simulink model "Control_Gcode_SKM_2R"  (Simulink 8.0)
settings: Solver=FixedStepDiscrete  SolverMode=SingleTasking  StartTime=0  StopTime=inf  FixedStep=dt  RelTol=1e-3  SampleTimeConstraint=Specified
InitFcn:
  | % Sampling Times %
  | dt0=0.001; dt1=0.01; samples=10;
undefined symbols (not defined in the file or in its folder): DiscIntNeverNeededParam, Volts
libraries: simulink_extras x4, speedgoatlib_IO311 x3, xpclib x3, speedgoatlib_IO101 x2, simulink x2

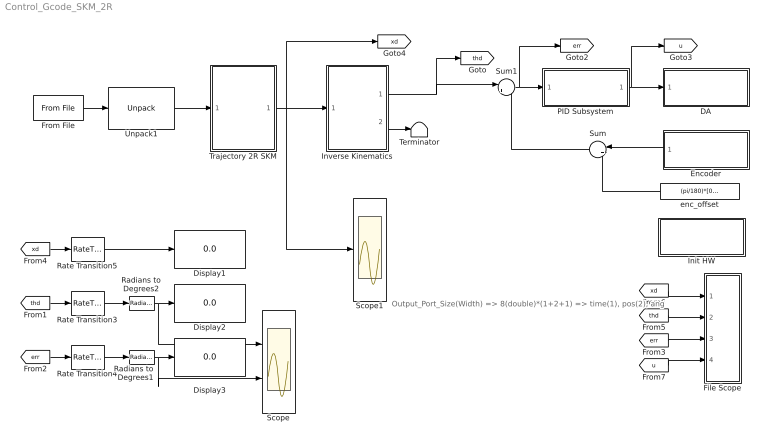
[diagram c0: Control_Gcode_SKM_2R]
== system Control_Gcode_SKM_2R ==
  note: Output_Port_Size(Width) => 8(double)*(1+2+1) => time(1), pos(2), ang
  DA : Subsystem  TreatAsAtomicUnit=on
  Display1 : Display
  Display2 : Display
  Display3 : Display
  Encoder : Subsystem  TreatAsAtomicUnit=on
  File Scope : Subsystem
  From File : xpclib/Misc./From File  filename='skm1.dat'  dataSize=32  bufSize=4000  readSize=1024  EOFOption=Hold last output  sampTime=dt0  show2ports=off
  Init HW : Subsystem  TreatAsAtomicUnit=on
  Inverse Kinematics : MATLAB Function  TreatAsAtomicUnit=on
  PID Subsystem : Subsystem  TreatAsAtomicUnit=on
  Radians to Degrees1 : simulink_extras/Transformations/Radians to Degrees
  Radians to Degrees2 : simulink_extras/Transformations/Radians to Degrees
  Rate Transition3 : RateTransition  OutPortSampleTime=dt1
  Rate Transition4 : RateTransition  OutPortSampleTime=dt1
  Rate Transition5 : RateTransition  OutPortSampleTime=dt1
  Scope : Scope  NumInputPorts=2
  Scope1 : Scope
  Sum : Sum  Inputs=|++
  Sum1 : Sum  Inputs=|+-
  Terminator : Terminator
  Trajectory 2R SKM : MATLAB Function  TreatAsAtomicUnit=on
  Unpack1 : xpclib/UDP/Unpack  dimensions={[4]}  datatypes={'double'}  byteAlign=1
  enc_offset : Constant  Value=(pi/180)*[0,90]'
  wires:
  [thd] -> Rate Transition3/1
  [err] -> Rate Transition4/1
  [xd] -> Rate Transition5/1
  Rate Transition5/1 -> Display1/1
  Rate Transition3/1 -> Radians to Degrees2/1
  Rate Transition4/1 -> Radians to Degrees1/1
  Radians to Degrees2/1 -> Display2/1, Scope/1
  Radians to Degrees1/1 -> Display3/1, Scope/2
  [xd] -> File Scope/1(xd)
  [thd] -> File Scope/2(thd)
  [err] -> File Scope/3(err)
  [u] -> File Scope/4(u)
  From File/1 -> Unpack1/1
  Sum1/1 -> PID Subsystem/1(In1), [err]
  PID Subsystem/1(Out1) -> DA/1(In1), [u]
  Encoder/1(Out1) -> Sum/1
  enc_offset/1 -> Sum/2
  Sum/1 -> Sum1/2
  Trajectory 2R SKM/1(xd) -> [xd], Inverse Kinematics/1(xd), Scope1/1
  Inverse Kinematics/1(thd) -> Sum1/1, [thd]
  Inverse Kinematics/2(w_index) -> Terminator/1
  Unpack1/1 -> Trajectory 2R SKM/1(traj)

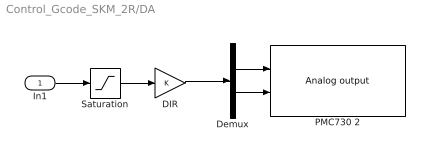
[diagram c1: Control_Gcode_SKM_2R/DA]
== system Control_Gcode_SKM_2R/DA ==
  In1 : Inport
  DIR : Gain
  Demux : Demux  Outputs=2
  PMC730 2 : speedgoatlib_IO101/Analog output  id=1  channel=[1,2]  reset=[1,1]  initValue=[0,0]  ts=dt0  pciSlot=-1
  Saturation : Saturate  UpperLimit=10  LowerLimit=-10
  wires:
  In1/1 -> Saturation/1
  Saturation/1 -> DIR/1
  DIR/1 -> Demux/1
  Demux/2 -> PMC730 2/2
  Demux/1 -> PMC730 2/1

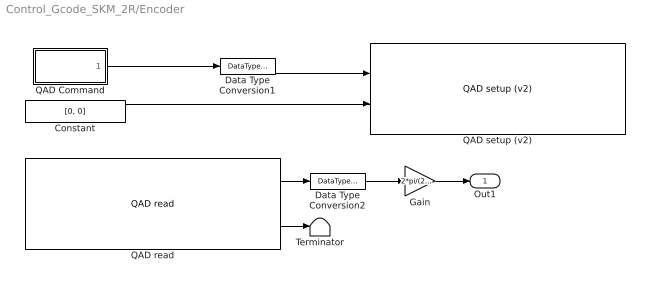
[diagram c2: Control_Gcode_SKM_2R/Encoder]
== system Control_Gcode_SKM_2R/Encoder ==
  Constant : Constant  Value=[0, 0]  OutDataTypeStr=Inherit: Inherit via back propagation
  Data Type Conversion1 : DataTypeConversion  OutDataTypeStr=uint8
  Data Type Conversion2 : DataTypeConversion  OutDataTypeStr=double
  Gain : Gain  Gain=2*pi/(23*2000)
  QAD Command : MATLAB Function  TreatAsAtomicUnit=on
  QAD read : speedgoatlib_IO311/QAD/QAD read  id=1  chan=[1 2]  pciSlot=-1  ts=dt0
  QAD setup (v2) : speedgoatlib_IO311/QAD/QAD setup (v2)  id=1  chan=[1,2]  debounce=0  quadrature=4x  index=Ignore index input  special=Disabled (cycling counter)  steps=2000  ts=dt0  pciSlot=-1
  Terminator : Terminator
  Out1 : Outport
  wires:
  Gain/1 -> Out1/1
  Constant/1 -> QAD setup (v2)/2
  QAD read/2 -> Terminator/1
  QAD read/1 -> Data Type Conversion2/1
  QAD Command/1(y) -> Data Type Conversion1/1
  Data Type Conversion2/1 -> Gain/1
  Data Type Conversion1/1 -> QAD setup (v2)/1

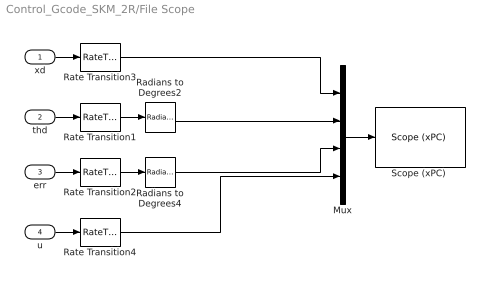
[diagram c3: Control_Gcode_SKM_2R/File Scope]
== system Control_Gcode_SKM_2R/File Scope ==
  xd : Inport
  thd : Inport  Port=2
  err : Inport  Port=3
  u : Inport  Port=4
  Mux : Mux
  Radians to Degrees2 : simulink_extras/Transformations/Radians to Degrees
  Radians to Degrees4 : simulink_extras/Transformations/Radians to Degrees
  Rate Transition{1..4} (4 alike) : RateTransition  OutPortSampleTime=dt1
  "Scope (xPC) " : xpclib/Misc./Scope (xPC)   scopeno=2  scopetype=File  autostart=on  viewmode=Graphical redraw  formatstr='%15.6f'  grid=on  ylimits=[0,0]  nosamples=100  noprepostsamples=0  interleave=1  triggermode=FreeRun  triggersignal=1  triggerlevel=0.0  triggerslope=Either  triggerscope=1  triggersample=0  filename=step3.dat  mode=Lazy  writesize=512  autorestart=on  dynamicfilemode=off  maxwritefilesize=512*1024^2
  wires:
  Radians to Degrees2/1 -> Mux/2
  Radians to Degrees4/1 -> Mux/3
  Rate Transition1/1 -> Radians to Degrees2/1
  Rate Transition2/1 -> Radians to Degrees4/1
  thd/1 -> Rate Transition1/1
  err/1 -> Rate Transition2/1
  Rate Transition3/1 -> Mux/1
  xd/1 -> Rate Transition3/1
  u/1 -> Rate Transition4/1
  Mux/1 -> "Scope (xPC) "/1
  Rate Transition4/1 -> Mux/4

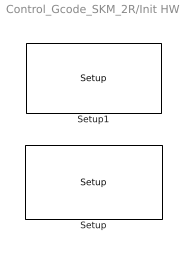
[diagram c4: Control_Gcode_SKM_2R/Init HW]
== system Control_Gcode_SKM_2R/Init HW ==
  Setup : speedgoatlib_IO311/Setup/Setup  group=Module setup  id=1  fpga1=speedgoat_IO311_default  pciSlot=-1  lowerDirection=[1 1 1 1 1 0 0 0 0 0 0 0 1 0 0 0]  lowerReset=[1]  lowerValue=[0]  upperDirection=[1 1 1 1 1 1 1 1 1 0 0 0 0 0 0 0]  upperReset=[1]  upperValue=[0]
  Setup1 : speedgoatlib_IO101/Setup  group=Module setup  id=1  pciSlot=-1  adStartChannel=1  adNumChannel=32  adCoupling=Single-ended  adRange=-10 .. 10 Volts  adAcqMode=Standard  daChannel=[1,2]  daReset=[1,1]  daInitValue=[0,0]  lowerChannel=1  lowerDirection=Input  lowerDIDebounce=0  lowerDOReset=[1]  lowerDOInitValues=[0]  upperChannel=1  upperDirection=Output  upperDIDebounce=0  upperDOReset=0  upperDOInitValues=0

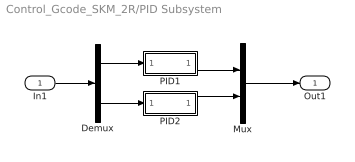
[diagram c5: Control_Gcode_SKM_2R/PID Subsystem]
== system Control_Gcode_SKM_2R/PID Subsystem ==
  In1 : Inport
  Demux : Demux  Outputs=2
  Mux : Mux  Inputs=2
  PID1 : Subsystem
  PID2 : Subsystem
  Out1 : Outport
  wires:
  In1/1 -> Demux/1
  Demux/1 -> PID1/1(In1)
  PID1/1(Out1) -> Mux/1
  Demux/2 -> PID2/1(In1)
  PID2/1(Out1) -> Mux/2
  Mux/1 -> Out1/1

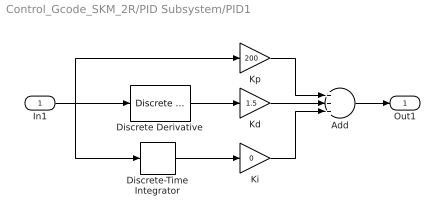
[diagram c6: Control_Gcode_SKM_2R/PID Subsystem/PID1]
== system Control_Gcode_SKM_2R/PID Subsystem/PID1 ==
  In1 : Inport
  Add : Sum  Inputs=+++
  Discrete Derivative : simulink/Discrete/Discrete Derivative  gainval=1.0  ICPrevScaledInput=0.0  InputProcessing=Inherited  OutMin=[]  OutMax=[]  OutDataType=fixdt(1, 16)  OutScaling=2^-10  DoSatur=off
  Discrete-Time Integrator : DiscreteIntegrator  SampleTime=dt0  ICPrevOutput=DiscIntNeverNeededParam  ICPrevScaledInput=DiscIntNeverNeededParam
  Kd : Gain  Gain=1.5
  Ki : Gain  Gain=0
  Kp : Gain  Gain=200
  Out1 : Outport
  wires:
  Discrete-Time Integrator/1 -> Ki/1
  Kp/1 -> Add/1
  Kd/1 -> Add/2
  Ki/1 -> Add/3
  Discrete Derivative/1 -> Kd/1
  Add/1 -> Out1/1
  In1/1 -> Kp/1, Discrete Derivative/1, Discrete-Time Integrator/1

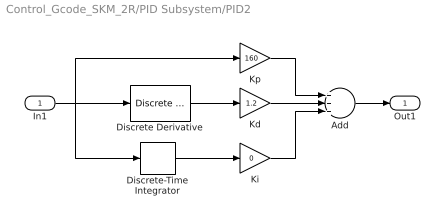
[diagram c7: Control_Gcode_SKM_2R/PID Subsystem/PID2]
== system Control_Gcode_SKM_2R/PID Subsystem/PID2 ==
  In1 : Inport
  Add : Sum  Inputs=+++
  Discrete Derivative : simulink/Discrete/Discrete Derivative  gainval=1.0  ICPrevScaledInput=0.0  InputProcessing=Inherited  OutMin=[]  OutMax=[]  OutDataType=fixdt(1, 16)  OutScaling=2^-10  DoSatur=off
  Discrete-Time Integrator : DiscreteIntegrator  SampleTime=dt0  ICPrevOutput=DiscIntNeverNeededParam  ICPrevScaledInput=DiscIntNeverNeededParam
  Kd : Gain  Gain=1.2
  Ki : Gain  Gain=0
  Kp : Gain  Gain=160
  Out1 : Outport
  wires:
  Discrete-Time Integrator/1 -> Ki/1
  Kp/1 -> Add/1
  Kd/1 -> Add/2
  Ki/1 -> Add/3
  Discrete Derivative/1 -> Kd/1
  Add/1 -> Out1/1
  In1/1 -> Kp/1, Discrete Derivative/1, Discrete-Time Integrator/1

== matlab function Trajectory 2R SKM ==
function xd = fcn(traj)

a1=100; a2=100;

x0=[a1,a2]';
xd=x0+traj(2:3,1);

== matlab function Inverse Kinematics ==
function [thd,w_index]  = fcn(xd)

persistent index thd_p

% Initializing Variables %
if isempty(index), index=0; end
if isempty(thd_p), thd_p=(pi/180)*[0,90]'; end

w_index=1;  % In workspace %
a1=100; a2=100;

% (1) Calculate th2 %
px=xd(1,1); py=xd(2,1);
kapha=(px^2+py^2-a1^2-a2^2)/(2*a1*a2);
if abs(kapha)>1
    w_index=-1;  % Out of Workspace %
    kapha=1;
end
th2=+acos(kapha); % Elbow Down %
%th2=-acos(kapha); % Elbow Up %
 
% (2) Calculate th1 %
delta=a1^2+a2^2+2*a1*a2*cos(th2);
cth1=(px*(a1+a2*cos(th2))+py*a2*sin(th2))/delta;
sth1=(-px*a2*sin(th2)+py*(a1+a2*cos(th2)))/delta;
th1=atan2(sth1, cth1);
if th1<0, th1=th1+2*pi; end % 0<th<360 %

% (3) Check Joint Limits %
if th1<0 || th1>pi, w_index=-1; end
if th2<pi/6 || th2>5*pi/6, w_index=-1; end

% Result %
if w_index==1
    thd=[th1, th2]';
else
    thd=thd_p;
end

% Save the current value %
thd_p=thd;

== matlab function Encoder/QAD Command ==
function y = fcn()

persistent index

if isempty(index), index=0; end

if index==0
    y=[1,1];      %  Reset %
else
    y = [0,0];
end

index=index+1;
